PROGRAM MAIN
VAR
	fbGetHostname : FB_GetHostName;
END_VAR

PRG_READ(); // Call sample for UA_Read
PRG_READ_List(); // Call sample for UA_ReadList
PRG_READ_List_Array(); // Call sample for UA_ReadList to read array elements
PRG_WRITE(); // Call sample for UA_Write
PRG_METHOD(); // Call sample for UA_MethodCall

END_PROGRAM
